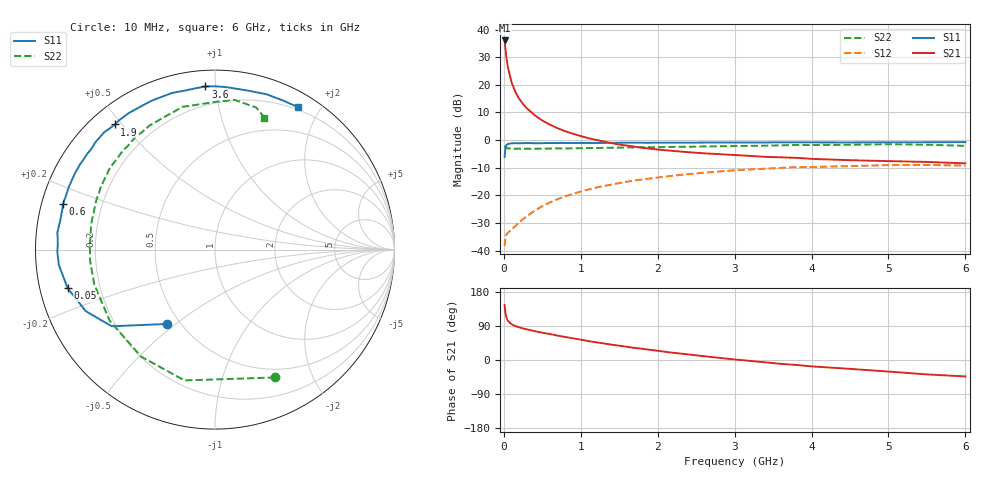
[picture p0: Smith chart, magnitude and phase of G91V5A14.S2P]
! SIEMENS Small Signal Semiconductors
! BFG235
! Si NPN RF Bipolar Junction Transistor in SOT223
! VCE = 1.5 V  IC = 140 mA
! Common Emitter S-Parameters:  July  1994
# GHz  S  MA  R  50
!  f  S11  S21  S12  S22
! GHz  MAG  ANG  MAG  ANG  MAG  ANG  MAG  ANG
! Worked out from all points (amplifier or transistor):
!   40 points, 10 MHz to 6 GHz, reference 50 ohm
!   highest |S21| = 36.1 dB at 10 MHz (marker M1)
!   |S21| within 3 dB of that: start of sweep to 20.31 MHz
!   unconditionally stable (mu >= 1): 402.5 MHz to 1.645 GHz; 1.745 GHz to 1.96 GHz
!   at 200 MHz: K = 0.82, MSG = 22.3 dB, |S12| = -29.8 dB
!   at 1.5 GHz: K = 1.01, MAG = 6.3 dB, |S12| = -15.6 dB
!   at 6 GHz: K = 0.94, MSG = 0.4 dB, |S12| = -9.2 dB
!   S11 on the Smith chart (normalised r, x): 10 MHz: 0.43, -0.47; 50 MHz: 0.08, -0.13; 600 MHz: 0.06, +0.15; 1.9 GHz: 0.07, +0.48; 3.6 GHz: 0.09, +0.94; 6 GHz: 0.17, +1.72
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0.01  0.4933 -122.9  63.59 145.2  0.012 54.5  0.7866 -64.9
0.02  0.7166 -143.4  45.44 125.2  0.0168 40.2  0.7484 -103.1
0.03  0.7973 -154.5  33.74 114.5  0.0191 34.3  0.7245 -124.6
0.05  0.8485 -165.3  21.57 104.1  0.0209 30.0  0.7082 -145.9
0.1  0.8743 -174.4  11.16 94.5  0.0239 35.7  0.7 -164.0
0.15  0.8788 -179.2  7.451 89.5  0.0278 43.1  0.6967 -171.5
0.2  0.8762 178.4  5.569 86.2  0.0325 48.1  0.6987 -175.6
0.25  0.8791 175.6  4.486 83.2  0.037 52.1  0.6962 -178.7
0.3  0.8835 173.8  3.748 80.9  0.0419 54.6  0.6979 178.7
0.4  0.877 169.7  2.822 76.1  0.0525 57.7  0.6967 175.0
0.5  0.8787 166.1  2.263 72.0  0.0634 59.0  0.7 171.8
0.6  0.8838 163.3  1.895 68.5  0.0744 59.3  0.7028 168.8
0.8  0.8863 156.8  1.442 60.6  0.0961 57.7  0.7053 163.5
1.1  0.8895 147.9  1.079 49.7  0.1274 53.6  0.7175 156.3
1.4  0.8884 140.7  0.882 40.4  0.1566 48.4  0.7267 149.7
1.9  0.8931 128.7  0.699 26.9  0.2018 39.1  0.7425 139.1
2.2  0.8999 122.2  0.636 19.0  0.2264 33.1  0.7529 133.2
3.2  0.9018 101.1  0.517 -2.4  0.2937 13.8  0.7845 114.4
3.6  0.9104 93.4  0.487 -10.2  0.3137 5.4  0.8021 106.3
4.5  0.9046 78.4  0.432 -23.4  0.3379 -10.0  0.8212 91.0
5.5  0.9132 65.4  0.402 -38.0  0.3552 -27.4  0.8242 73.8
6  0.9178 59.9  0.379 -43.4  0.3451 -33.9  0.7856 69.5
